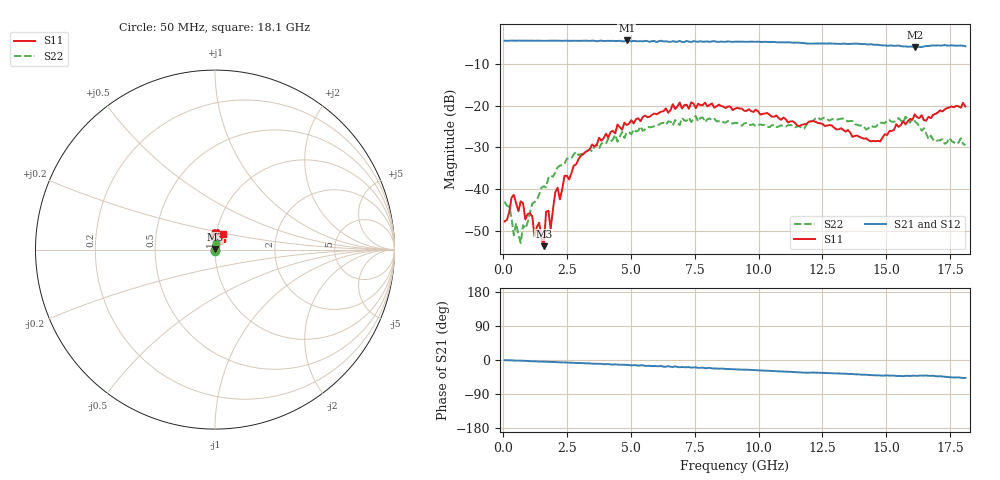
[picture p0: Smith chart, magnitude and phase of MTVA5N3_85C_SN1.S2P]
! Network Analyzer HP8720D.06.14 Serial No. US36140669
! 11 May 2005  11:45:11
! Frequency  S11  S21  S12  S22
# HZ  S  DB R 50
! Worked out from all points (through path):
!   201 points, 50 MHz to 18.1 GHz, reference 50 ohm
!   highest |S21| = -4.36 dB at 4.833 GHz (marker M1); lowest = -6.0 dB at 16.11 GHz (marker M2)
!   group delay of S21, straight-line fit = 7.31 ps
!   lowest |S11| = -53.7 dB at 1.584 GHz (marker M3), VSWR 1.00, Z = 50.1 + j0.197 ohm
!   |S11| at or under -10 dB: start of sweep to end of sweep
!   |S22| runs from -52.9 to -22.5 dB; largest |S21 - S12| = 0.021
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5e7  -47.77 -66.5  -4.42 -0.4  -4.44 -0.7  -43.02 -69.9
4.11e8  -41.38 -155.7  -4.43 -1.2  -4.42 -1.7  -51.09 1.0
5.0125e8  -43.46 -142.5  -4.44 -1.6  -4.41 -1.9  -48.19 5.0
6.8175e8  -42.95 -175.8  -4.42 -1.9  -4.42 -2.3  -52.92 44.0
1.133e9  -46.58 -176.3  -4.42 -3.3  -4.43 -3.6  -43.50 81.4
1.22325e9  -51.40 174.4  -4.45 -3.3  -4.43 -3.8  -43.13 76.1
1.40375e9  -48.07 153.4  -4.42 -3.9  -4.42 -4.2  -41.26 91.9
1.58425e9  -53.70 72.6  -4.43 -4.4  -4.43 -4.7  -39.34 85.3
1.6745e9  -45.47 83.3  -4.42 -4.5  -4.42 -4.9  -39.60 87.8
1.855e9  -49.54 97.2  -4.44 -5.1  -4.43 -5.4  -36.76 88.0
2.0355e9  -40.76 64.1  -4.43 -5.5  -4.43 -5.9  -36.04 92.4
2.216e9  -42.47 73.0  -4.44 -6.0  -4.41 -6.4  -34.38 85.0
2.3965e9  -36.84 58.5  -4.44 -6.4  -4.43 -6.8  -33.99 90.3
3.1185e9  -31.69 63.4  -4.44 -8.2  -4.45 -8.8  -31.52 111.5
4.83325e9  -24.65 76.5  -4.36 -12.8  -4.45 -13.8  -26.41 86.5
6.09675e9  -21.74 78.4  -4.52 -16.4  -4.47 -16.8  -24.55 81.5
9.075e9  -20.75 97.1  -4.65 -24.4  -4.62 -24.8  -24.11 67.5
1.21435e10  -23.68 102.7  -5.11 -33.0  -5.07 -33.5  -23.62 76.4
1.439975e10  -28.57 54.8  -5.27 -39.9  -5.25 -40.1  -24.83 76.6
1.512175e10  -26.08 48.9  -5.61 -41.2  -5.50 -41.2  -23.50 78.2
1.61145e10  -22.09 42.5  -5.97 -41.4  -5.78 -42.0  -23.71 62.8
1.81e10  -20.21 62.6  -5.78 -47.1  -5.77 -48.2  -29.50 78.6
